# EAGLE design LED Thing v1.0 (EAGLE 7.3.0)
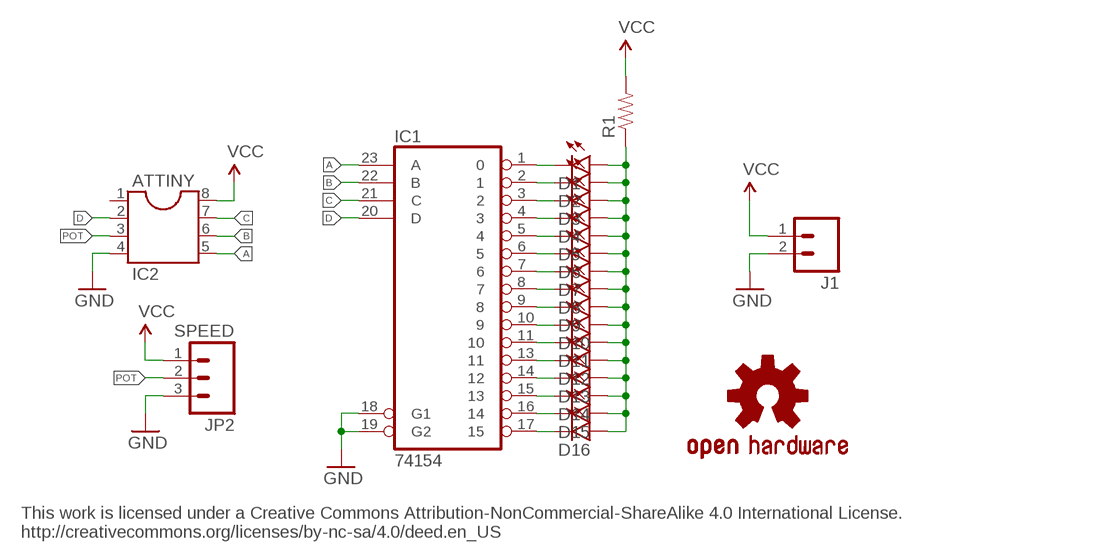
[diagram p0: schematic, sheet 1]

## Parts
ATTINY  IC2  DIL8  [DIL08]
D1  LED-RED1206  [LED-1206]
D2  LED-RED1206  [LED-1206]
D3  LED-RED1206  [LED-1206]
D4  LED-RED1206  [LED-1206]
D5  LED-RED1206  [LED-1206]
D6  LED-RED1206  [LED-1206]
D7  LED-RED1206  [LED-1206]
D8  LED-RED1206  [LED-1206]
D9  LED-RED1206  [LED-1206]
D10  LED-RED1206  [LED-1206]
D11  LED-RED1206  [LED-1206]
D12  LED-RED1206  [LED-1206]
D13  LED-RED1206  [LED-1206]
D14  LED-RED1206  [LED-1206]
D15  LED-RED1206  [LED-1206]
D16  LED-RED1206  [LED-1206]
IC1  74154  74HC154N  [DIL24-6]
J1  M02PTH  [1X02]
JP2  SPEED  M031X03_NO_SILK  [1X03_NO_SILK]
LOGO2  OSHW-LOGOM  [OSHW-LOGO-M]
R1  RESISTOR0805-RES  [0805]

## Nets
A: ATTINY.5 IC1.23(A)
B: ATTINY.6 IC1.22(B)
C: ATTINY.7 IC1.21(C)
D: ATTINY.2 IC1.20(D)
GND: ATTINY.4 IC1.18(G1) IC1.19(G2) J1.2 JP2.3
N$1: D1.C IC1.1
N$2: D2.C IC1.2
N$3: D3.C IC1.3
N$4: D4.C IC1.4
N$5: D5.C IC1.5
N$6: D6.C IC1.6
N$7: D7.C IC1.7
N$8: D8.C IC1.8
N$9: D9.C IC1.9
N$10: D10.C IC1.10
N$11: D11.C IC1.11
N$12: D12.C IC1.13
N$13: D13.C IC1.14
N$14: D14.C IC1.15
N$15: D15.C IC1.16
N$16: D16.C IC1.17
N$17: D1.A D2.A D3.A D4.A D5.A D6.A D7.A D8.A D9.A D10.A D11.A D12.A D13.A D14.A D15.A D16.A R1.1
POT: ATTINY.3 JP2.2
VCC: ATTINY.8 J1.1 JP2.1 R1.2
Unconnected: ATTINY.1

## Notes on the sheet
- This work is licensed under a Creative Commons Attribution-NonCommercial-ShareAlike 4.0 International License.
  http://creativecommons.org/licenses/by-nc-sa/4.0/deed.en_US

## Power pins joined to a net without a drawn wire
GND: IC1.12(GND)
VCC: IC1.24(VCC)

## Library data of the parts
ATTINY = ic-package:DIL8: Dual In Line / Socket
D1-D16 = SparkFun-LED:LED-RED: Assorted Red LEDs; PROD_ID: DIO-00809; VALUE: RED
IC1 = 74xx-eu:74*154: 4-line to 16-line data SELECTOR/MULTIPLEXER
J1 = SparkFun-Connectors:M02: Standard 2-pin 0.1" header. Use with
JP2 = SparkFun-Connectors:M03: Header 3 Standard 3-pin 0.1" header. Use with straight break away headers (SKU : PRT-00116), right angle break away headers (PRT-00553), swiss pins (PRT-00743), machine pins (PRT-00117), and female headers (PRT-00115). Molex polarized connector foot print use with SKU : PRT-08232 with associated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
LOGO2 = SparkFun-Aesthetics:OSHW-LOGO: Open Source Hardware Logo
R1 = SparkFun-Resistors:RESISTOR: Resistor

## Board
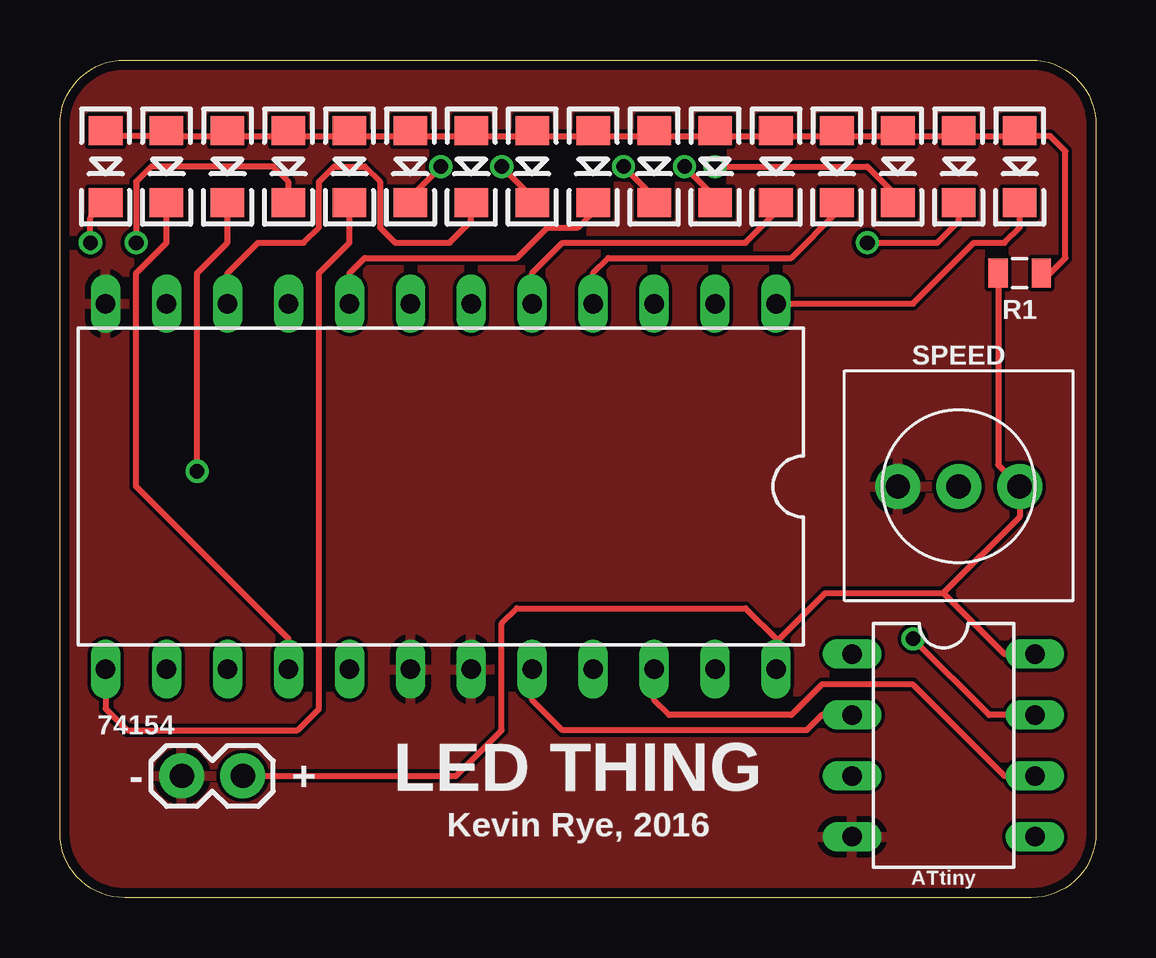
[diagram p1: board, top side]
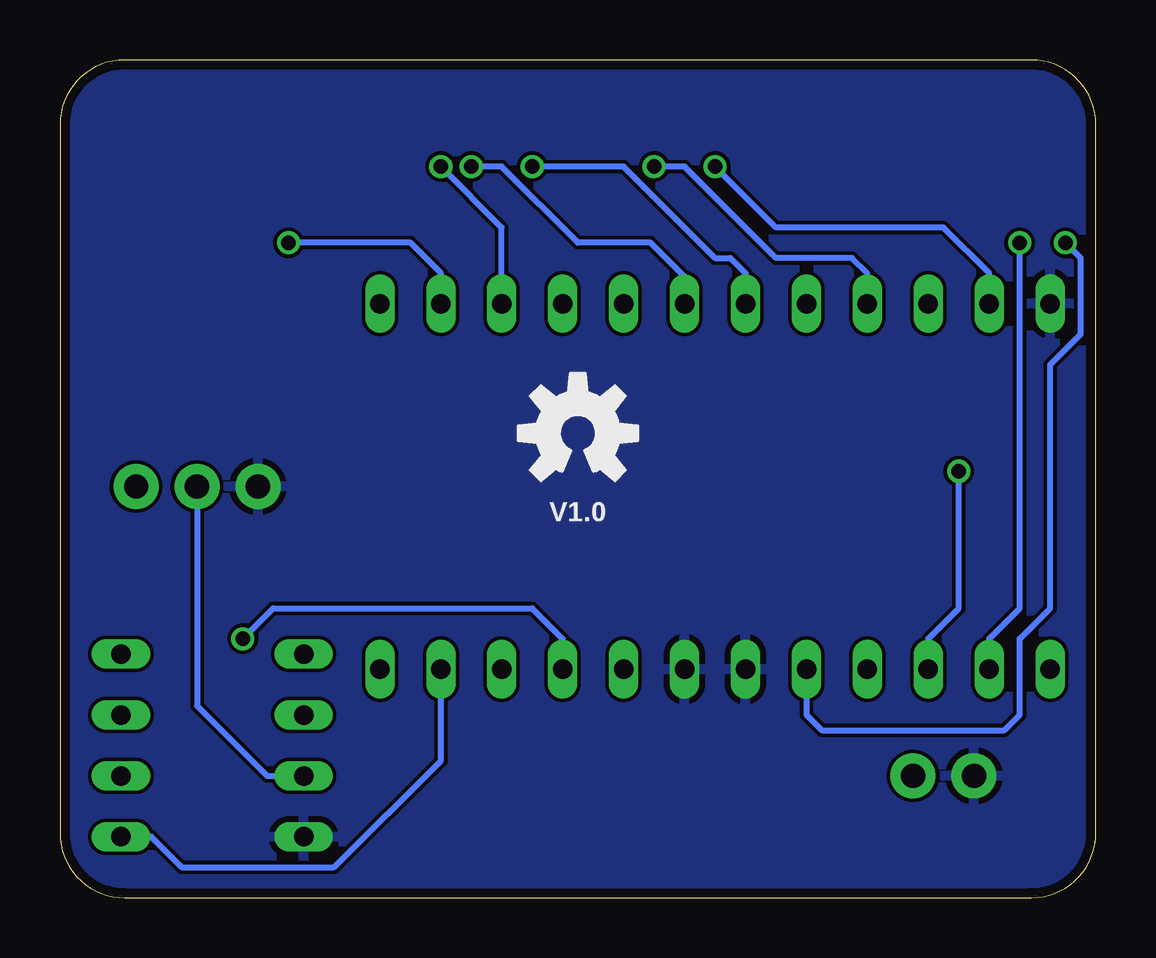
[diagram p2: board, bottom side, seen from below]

Size 43.18 x 34.92 mm. Coordinates in mm from the lower left corner, seen from the top.
Outline: 40.49,34.92 arc-90 43.18,32.23 43.18,2.69 arc-90 40.49,0 2.69,0 arc-90 0,2.69 0,32.23 arc-90 2.69,34.92 40.49,34.92
Copper layers (1*16): Top 0.0356mm / dielectric 1.5011mm / Bottom 0.0356mm
Design rules "oshpark-2layer": minimum track width 6mil, minimum drill 13mil, track to track 6mil, track to pad 6mil, pad to pad 6mil, via to via 6mil, smd to smd 6mil, copper to edge 15mil, drill to drill 6mil, minimum pad ring 7mil, minimum via ring 7mil, stop-mask expansion 2.5mil, vias tented up to drill 0mil, thermal gap 10mil

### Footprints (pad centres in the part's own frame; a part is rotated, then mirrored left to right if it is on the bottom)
DIL08 = drill 0.813 long: 1 -3.81,-3.81; 2 -1.27,-3.81; 3 1.27,-3.81; 4 3.81,-3.81; 5 3.81,3.81; 6 1.27,3.81; 7 -1.27,3.81; 8 -3.81,3.81
LED-1206 = smd 1.2 x 1.4: A -1.5,0; C 1.5,0
DIL24-6 = drill 0.813 long: 1 -13.97,-7.62; 2 -11.43,-7.62; 3 -8.89,-7.62; 4 -6.35,-7.62; 5 -3.81,-7.62; 6 -1.27,-7.62; 7 1.27,-7.62; 8 3.81,-7.62; 9 6.35,-7.62; 10 8.89,-7.62; 11 11.43,-7.62; 12 13.97,-7.62; 13 13.97,7.62; 14 11.43,7.62; 15 8.89,7.62; 16 6.35,7.62; 17 3.81,7.62; 18 1.27,7.62; 19 -1.27,7.62; 20 -3.81,7.62; 21 -6.35,7.62; 22 -8.89,7.62; 23 -11.43,7.62; 24 -13.97,7.62
1X02 = drill 1.016 pad 1.88: 1 0,0; 2 2.54,0
1X03_NO_SILK = drill 1.016 pad 1.88: 1 0,0; 2 2.54,0; 3 5.08,0
0805 = smd 0.8 x 1.2: 1 -0.9,0; 2 0.9,0

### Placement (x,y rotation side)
ATTINY  36.83,6.35 270 top
D1  40.01,30.48 270 top
D2  37.47,30.48 270 top
D3  34.92,30.48 270 top
D4  32.38,30.48 270 top
D5  29.84,30.48 270 top
D6  27.3,30.48 270 top
D7  24.77,30.48 270 top
D8  22.23,30.48 270 top
D9  19.68,30.48 270 top
D10  17.14,30.48 270 top
D11  14.61,30.48 270 top
D12  12.06,30.48 270 top
D13  9.53,30.48 270 top
D14  6.99,30.48 270 top
D15  4.45,30.48 270 top
D16  1.91,30.48 270 top
IC1  15.88,17.14 180 top
J1  7.62,5.08 180 top
JP2  40.01,17.14 180 top
LOGO2  21.59,19.37 0 bottom
R1  40.01,26.04 180 top

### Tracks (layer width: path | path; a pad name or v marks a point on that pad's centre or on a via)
A
  Bottom 0.254: IC1.23 27.3,5.71 31.75,1.27 38.1,1.27 39.37,2.54 ATTINY.5
B
  Top 0.254: IC1.22 24.77,8.26 25.4,7.62 30.48,7.62 31.75,8.89 35.56,8.89 39.37,5.08 ATTINY.6
C  (via drill 0.61)
  Top 0.254: v35.56,10.79 38.73,7.62 ATTINY.7
  Bottom 0.254: IC1.21 22.23,10.79 23.5,12.06 34.29,12.06 v35.56,10.79
D
  Top 0.254: ATTINY.2 31.75,7.62 31.11,6.99 20.95,6.99 19.68,8.26 IC1.20
GND
  pour Top: -1.27,-1.91 44.45,-1.91 44.45,36.2 -1.27,36.2
  pour Bottom: -0.64,-1.27 -0.64,35.56 43.81,36.2 43.81,-1.27
N$1
  Top 0.254: IC1.1 35.56,24.77 38.1,27.3 39.37,27.3 40.01,27.94 D1.C
N$2  (via drill 0.61)
  Top 0.254: v33.66,27.3 36.57,27.3 37.47,28.2 D2.C
  Bottom 0.254: v33.66,27.3 28.57,27.3 27.3,26.04 IC1.2
N$3  (via drill 0.61)
  Top 0.254: v27.3,30.48 33.66,30.48 34.92,29.21 D3.C
  Bottom 0.254: v27.3,30.48 24.77,27.94 IC1.3
N$4
  Top 0.254: IC1.4 22.23,26.04 22.86,26.67 30.48,26.67 32.38,28.57 D4.C
N$5
  Top 0.254: IC1.5 19.68,26.04 20.95,27.3 28.57,27.3 29.84,28.57 D5.C
N$6  (via drill 0.61)
  Top 0.254: v26.04,30.48 27.3,29.21 D6.C
  Bottom 0.254: v26.04,30.48 24.77,30.48 21.59,27.3 18.57,27.3 17.14,25.89 IC1.6
N$7  (via drill 0.61)
  Top 0.254: v23.5,30.48 24.77,29.21 D7.C
  Bottom 0.254: v23.5,30.48 19.68,30.48 15.88,26.67 15.24,26.67 14.61,26.04 IC1.7
N$8
  Top 0.254: IC1.8 12.06,26.04 12.7,26.67 19.05,26.67 20.32,27.94 21.59,27.94 22.23,28.57 D8.C
N$9  (via drill 0.61)
  Top 0.254: v18.41,30.48 19.68,29.21 D9.C
  Bottom 0.254: v18.41,30.48 17.14,30.48 13.34,26.67 10.16,26.67 9.53,26.04 IC1.9
N$10
  Top 0.254: D10.C 17.14,28.2 16.25,27.3 13.97,27.3 13.34,27.94 13.34,29.84 12.7,30.48 11.43,30.48 10.79,29.84 10.79,27.94 10.16,27.3 8.26,27.3 6.99,26.04 IC1.10
N$11  (via drill 0.61)
  Top 0.254: v15.88,30.48 14.61,29.21 D11.C
  Bottom 0.254: v15.88,30.48 13.34,27.94 6.35,27.94 4.45,26.04 IC1.11
N$12
  Top 0.254: D12.C 12.06,27.3 10.79,26.04 10.79,7.88 9.9,6.99 2.8,6.99 1.91,7.88 IC1.13
N$13  (via drill 0.61)
  Top 0.254: 9.53,29.21 D13.C 9.53,29.84 8.89,30.48 3.81,30.48 3.17,29.84 v3.17,27.3
  Bottom 0.254: v3.17,27.3 3.17,12.06 4.45,10.79 IC1.14
N$14  (via drill 0.61)
  Top 0.254: D14.C 6.99,27.3 5.71,26.04 v5.71,17.78
  Bottom 0.254: v5.71,17.78 5.71,12.06 6.99,10.79 IC1.15
N$15
  Top 0.254: D15.C 4.45,27.3 3.17,26.04 3.17,17.14 9.53,10.79 IC1.16
N$16  (via drill 0.61)
  Top 0.254: v1.27,27.3 1.27,28.34 D16.C
  Bottom 0.254: IC1.17 12.06,7.62 11.43,6.99 3.81,6.99 3.17,7.62 3.17,10.79 1.91,12.06 1.91,22.23 0.64,23.5 0.64,26.67 v1.27,27.3
N$17
  Top 0.254: 4.45,31.75 1.91,31.75 D16.A | 4.45,31.75 6.99,31.75 | 4.45,31.75 D15.A | 6.99,31.75 9.53,31.75 | 6.99,31.75 D14.A | 9.53,31.75 12.06,31.75 | 9.53,31.75 D13.A | 12.06,31.75 14.61,31.75 | 12.06,31.75 D12.A | 14.61,31.75 17.14,31.75 | 14.61,31.75 D11.A | 17.14,31.75 19.68,31.75 | 17.14,31.75 D10.A | 19.68,31.75 22.23,31.75 | 19.68,31.75 D9.A | 22.23,31.75 24.77,31.75 | 22.23,31.75 D8.A | 24.77,31.75 27.3,31.75 | 24.77,31.75 D7.A | 27.3,31.75 29.84,31.75 | 27.3,31.75 D6.A | 29.84,31.75 32.38,31.75 | 29.84,31.75 D5.A | 32.38,31.75 34.92,31.75 | 32.38,31.75 D4.A | 34.92,31.75 37.47,31.75 | 34.92,31.75 D3.A | 37.47,31.75 40.01,31.75 D1.A 40.23,31.75 41.27,31.75 41.91,31.11 41.91,26.67 40.91,25.66 R1.1 | 37.47,31.75 D2.A
POT
  Bottom 0.254: JP2.2 37.47,8.01 34.54,5.08 ATTINY.3
VCC
  Top 0.254: 29.92,10.72 31.9,12.7 36.83,12.7 | 29.92,10.72 29.84,10.64 IC1.24 | 36.83,12.7 39.37,10.16 ATTINY.8 | 36.83,12.7 40.01,15.88 JP2.1 39.1,18.05 R1.2 | J1.1 16.51,5.08 18.41,6.99 18.41,11.43 19.05,12.06 28.57,12.06 29.92,10.72

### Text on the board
Unrouted: This work is licensed under a Creative Commons Attribution-NonCommercial-ShareAlike 4.0 International License. / http://creativecommons.org/licenses/by-nc-sa/4.0/deed.en_US
tPlace: LED THING | Kevin Rye, 2016 | ATtiny
bPlace: V1.0
tNames: - | +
